| TEXAS INSTRUMENTS INCORPORATED
| Standard Linear and Logic Group
| IBIS Model of SN74AUC16373
| 16-BIT TRANSPARENT D-TYPE LATCH WITH 3-STATE OUTPUTS
| This file contains package information for the following:
|  TSSOP 48-pin (DGG) package as [Component] AUC16373_DGG
|   TVSOP 48-pin (DGV) package as [Component] AUC16373_DGV
|   VFBGA 56-pin (GQL) package as [Component] AUC16373_GQL
| This device can be powered at the following Vccs:
|  2.5 volt Vcc
|  1.8 volt Vcc
|  1.5 volt Vcc
|  1.2 volt Vcc
|  0.8 volt Vcc
| This file provides unique models under the [Model Selector] for each Vcc.
| For operation at a specific Vcc, select the appropriate model after each
| [Model Selector] keyword.
[IBIS Ver]   3.2
[Comment char]  |_char
[File Name]   sn74auc16373.ibs
[File Rev]   1.1 | x_die
[Date]   June 20, 2002
[Source]   Data created from TI-SPICE simulations at TI-SLL.
[Notes]   The following is an IBIS list for the AUC16373.
   Please contact sllibis@ti.com with questions and
   comments concerning SLL IBIS models.
   -The waveforms for the AUC16373_OUT Power Clamp ,Pullup, and
   Pulldown are caused by the circuitry that helps reduce
   overshoot and undershoot in transmission lines (EMI).
   These waveforms are norimal for this particular design.
   -Power clamp data deleted as there is no power-clamp diode.
   -End point warning due to AC and DC mismatch.
[Disclaimer] Property of Texas Instruments Incorporated.  Unauthorized
   reproduction and/or distribution is strictly prohibited.
   This product is protected under copyright law.
   Created  2002, (C) Copyright  2002, Texas Instruments
   Incorporated, All Rights Reserved
   UNLESS THERE IS A SIGNED, WRITTEN AGREEMENT TO THE
   CONTRARY, TEXAS INSTRUMENTS (TI) IS PROVIDING THE IBIS
   MODELS  AND WITHOUT ANY WARRANTY, EXPRESSED OR
   IMPLIED.  TI assumes no liability for:
   1) the accuracy of the IBIS models provided to your
   company;
   2) the proper functioning of these IBIS Models in your
   design or for any resulting applications; or
   3) infringement of patents, copyrights or intellectual
   property rights resulting from your use of these IBIS
   models.
   TI provides IBIS Models as a service to our customers.
   You and your company shall not distribute, sell or give
   these models to anyone else without prior written
   permission from TI.
   TI reserves the right to make changes to our products or
   to discontinue any semiconductor product or service
   without notice, and advises our customers to obtain the
   latest version of relevant information to verify, before
   placing orders, that the information being relied on is
   current.
   Please be aware that your receipt and use of the IBIS
   information provided shall serve as acceptance of these
   terms and conditions.  If you do not accept these terms,
   you should return or destroy the IBIS models and any
   other accompanying information immediately.
| Component AUC16373_DGG 48-pin TSSOP
[Component]   AUC16373_DGG
[Manufacturer]   Texas Instruments, Inc.
[Package]
|   typ   min   max
R_pkg   6.200e-02   5.000e-02   7.800e-02
L_pkg   3.527e-09   3.128e-09   4.255e-09
C_pkg   5.300e-13   4.170e-13   6.850e-13
[Pin]   signal_name   model_name   R_pin   L_pin   C_pin
1   1NOE   AUC16373_OEIN   5.000e-02   4.250e-09   6.710e-13
2   1Q1   AUC16373_OUT   5.700e-02   3.956e-09   6.740e-13
3   1Q2   AUC16373_OUT   7.100e-02   3.922e-09   6.190e-13
4   GND   GND   7.800e-02   3.841e-09   6.180e-13
5   1Q3   AUC16373_OUT   5.600e-02   3.535e-09   5.550e-13
6   1Q4   AUC16373_OUT   5.800e-02   3.464e-09   5.030e-13
7   VCC   POWER   6.000e-02   3.362e-09   4.980e-13
8   1Q5   AUC16373_OUT   6.100e-02   3.293e-09   4.620e-13
9   1Q6   AUC16373_OUT   6.300e-02   3.240e-09   4.550e-13
10   GND   GND   6.300e-02   3.175e-09   4.420e-13
11   1Q7   AUC16373_OUT   6.400e-02   3.153e-09   4.290e-13
12   1Q8   AUC16373_OUT   6.500e-02   3.128e-09   4.180e-13
13   2Q1   AUC16373_OUT   6.500e-02   3.128e-09   4.180e-13
14   2Q2   AUC16373_OUT   6.400e-02   3.154e-09   4.290e-13
15   GND   GND   6.300e-02   3.174e-09   4.420e-13
16   2Q3   AUC16373_OUT   6.300e-02   3.241e-09   4.550e-13
17   2Q4   AUC16373_OUT   6.100e-02   3.293e-09   4.620e-13
18   VCC   POWER   6.000e-02   3.362e-09   4.970e-13
19   2Q5   AUC16373_OUT   5.800e-02   3.464e-09   5.030e-13
20   2Q6   AUC16373_OUT   5.600e-02   3.537e-09   5.600e-13
21   GND   GND   7.700e-02   3.839e-09   6.260e-13
22   2Q7   AUC16373_OUT   7.100e-02   3.917e-09   6.270e-13
23   2Q8   AUC16373_OUT   5.800e-02   3.955e-09   6.850e-13
24   2NOE   AUC16373_OEIN   5.200e-02   4.255e-09   6.790e-13
25   2LE   AUC16373_LEIN   5.100e-02   4.254e-09   6.760e-13
26   2D8   AUC16373_IN   5.800e-02   3.957e-09   6.790e-13
27   2D7   AUC16373_IN   7.100e-02   3.920e-09   6.210e-13
28   GND   GND   7.800e-02   3.843e-09   6.220e-13
29   2D6   AUC16373_IN   5.600e-02   3.539e-09   5.600e-13
30   2D5   AUC16373_IN   5.800e-02   3.466e-09   5.030e-13
31   VCC   POWER   6.000e-02   3.363e-09   4.970e-13
32   2D4   AUC16373_IN   6.100e-02   3.294e-09   4.620e-13
33   2D3   AUC16373_IN   6.300e-02   3.241e-09   4.540e-13
34   GND   GND   6.300e-02   3.175e-09   4.410e-13
35   2D2   AUC16373_IN   6.400e-02   3.153e-09   4.290e-13
36   2D1   AUC16373_IN   6.500e-02   3.129e-09   4.170e-13
37   1D8   AUC16373_IN   6.500e-02   3.129e-09   4.170e-13
38   1D7   AUC16373_IN   6.400e-02   3.152e-09   4.290e-13
39   GND   GND   6.400e-02   3.176e-09   4.410e-13
40   1D6   AUC16373_IN   6.300e-02   3.241e-09   4.540e-13
41   1D5   AUC16373_IN   6.100e-02   3.293e-09   4.620e-13
42   VCC   POWER   6.000e-02   3.363e-09   4.970e-13
43   1D4   AUC16373_IN   5.800e-02   3.464e-09   5.030e-13
44   1D3   AUC16373_IN   5.600e-02   3.534e-09   5.610e-13
45   GND   GND   7.800e-02   3.841e-09   6.260e-13
46   1D2   AUC16373_IN   7.100e-02   3.920e-09   6.220e-13
47   1D1   AUC16373_IN   5.700e-02   3.955e-09   6.770e-13
48   1LE   AUC16373_LEIN   5.100e-02   4.252e-09   6.720e-13
| Component AUC16373_DGV 48-pin TVSOP
[Component]   AUC16373_DGV
[Manufacturer]   Texas Instruments, Inc.
[Package]
|   typ   min   max
R_pkg   7.000e-02   4.900e-02   8.500e-02
L_pkg   3.013e-09   2.743e-09   3.408e-09
C_pkg   3.710e-13   2.940e-13   5.110e-13
[Pin]   signal_name   model_name   R_pin   L_pin   C_pin
1   1NOE   AUC16373_OEIN   4.900e-02   3.393e-09   4.970e-13
2   1Q1   AUC16373_OUT   6.000e-02   3.250e-09   5.020e-13
3   1Q2   AUC16373_OUT   7.700e-02   3.310e-09   4.510e-13
4   GND   GND   8.500e-02   3.299e-09   4.040e-13
5   1Q3   AUC16373_OUT   8.300e-02   3.136e-09   3.600e-13
6   1Q4   AUC16373_OUT   7.700e-02   3.019e-09   3.630e-13
7   VCC   POWER   6.500e-02   2.882e-09   3.490e-13
8   1Q5   AUC16373_OUT   6.600e-02   2.829e-09   3.140e-13
9   1Q6   AUC16373_OUT   6.700e-02   2.796e-09   3.140e-13
10   GND   GND   6.900e-02   2.754e-09   3.080e-13
11   1Q7   AUC16373_OUT   7.000e-02   2.753e-09   3.010e-13
12   1Q8   AUC16373_OUT   7.100e-02   2.745e-09   2.940e-13
13   2Q1   AUC16373_OUT   7.000e-02   2.744e-09   2.940e-13
14   2Q2   AUC16373_OUT   7.000e-02   2.754e-09   3.010e-13
15   GND   GND   6.900e-02   2.754e-09   3.080e-13
16   2Q3   AUC16373_OUT   6.700e-02   2.796e-09   3.140e-13
17   2Q4   AUC16373_OUT   6.600e-02   2.829e-09   3.140e-13
18   VCC   POWER   6.500e-02   2.883e-09   3.500e-13
19   2Q5   AUC16373_OUT   7.500e-02   3.014e-09   3.630e-13
20   2Q6   AUC16373_OUT   8.000e-02   3.128e-09   3.580e-13
21   GND   GND   8.400e-02   3.295e-09   4.030e-13
22   2Q7   AUC16373_OUT   7.800e-02   3.311e-09   4.520e-13
23   2Q8   AUC16373_OUT   6.200e-02   3.259e-09   5.010e-13
24   2NOE   AUC16373_OEIN   5.200e-02   3.404e-09   4.960e-13
25   2LE   AUC16373_OEIN   5.300e-02   3.397e-09   5.050e-13
26   2D8   AUC16373_IN   6.200e-02   3.249e-09   5.110e-13
27   2D7   AUC16373_IN   7.700e-02   3.308e-09   4.530e-13
28   GND   GND   8.200e-02   3.289e-09   4.030e-13
29   2D6   AUC16373_IN   7.800e-02   3.121e-09   3.590e-13
30   2D5   AUC16373_IN   7.400e-02   3.010e-09   3.630e-13
31   VCC   POWER   6.500e-02   2.883e-09   3.490e-13
32   2D4   AUC16373_IN   6.700e-02   2.829e-09   3.140e-13
33   2D3   AUC16373_IN   6.700e-02   2.795e-09   3.140e-13
34   GND   GND   6.900e-02   2.753e-09   3.070e-13
35   2D2   AUC16373_IN   7.000e-02   2.753e-09   3.010e-13
36   2D1   AUC16373_IN   7.000e-02   2.743e-09   2.940e-13
37   1D8   AUC16373_IN   7.000e-02   2.743e-09   2.940e-13
38   1D7   AUC16373_IN   7.000e-02   2.753e-09   3.010e-13
39   GND   GND   6.900e-02   2.754e-09   3.070e-13
40   1D6   AUC16373_IN   6.800e-02   2.797e-09   3.140e-13
41   1D5   AUC16373_IN   6.700e-02   2.830e-09   3.140e-13
42   VCC   POWER   6.400e-02   2.880e-09   3.490e-13
43   1D4   AUC16373_IN   7.200e-02   3.004e-09   3.620e-13
44   1D3   AUC16373_IN   7.800e-02   3.121e-09   3.590e-13
45   GND   GND   8.400e-02   3.296e-09   4.030e-13
46   1D2   AUC16373_IN   7.700e-02   3.308e-09   4.510e-13
47   1D1   AUC16373_IN   6.200e-02   3.258e-09   4.990e-13
48   1LE   AUC16373_OEIN   5.300e-02   3.408e-09   4.940e-13
|   VFBGA PACKAGE (GQL)
[Component]   AUC16373_GQL
[manufacturer]   Texas Instruments, Inc.
[Package]
|   typ   min   max
R_pkg   0.065   0.035   0.097
L_pkg   1.952nH   1.000nH   3.191nH
C_pkg   0.283pF   0.162pF   0.434pF
[Pin] signal_name   model_name   R_pin   L_pin   C_pin
A3   NC   NC   0.036   1.004nH   0.176pF
A2   NC   NC   0.04   1.191nH   0.186pF
A1   1NOE   AUC16373_OEIN   0.047   1.411nH   0.209pF
B3   GND   GND   0.097   3.191nH   0.434pF
B2   1Q1   AUC16373_OUT   0.074   2.213nH   0.329pF
B1   1Q2   AUC16373_OUT   0.06   1.712nH   0.243pF
C3   VCC   POWER   0.085   2.691nH   0.368pF
C2   1Q3   AUC16373_OUT   0.074   2.16nH   0.315pF
C1   1Q4   AUC16373_OUT   0.06   1.666nH   0.247pF
D2   1Q5   AUC16373_OUT   0.074   2.121nH   0.313pF
D3   GND   GND   0.091   2.924nH   0.397pF
D1   1Q6   AUC16373_OUT   0.06   1.619nH   0.245pF
E2   1Q7   AUC16373_OUT   0.069   2.031nH   0.288pF
E1   1Q8   AUC16373_OUT   0.06   1.583nH   0.22pF
F1   2Q1   AUC16373_OUT   0.06   1.578nH   0.22pF
F2   2Q2   AUC16373_OUT   0.069   2.017nH   0.286pF
G1   2Q3   AUC16373_OUT   0.06   1.594nH   0.241pF
G3   GND   GND   0.092   2.917nH   0.397pF
G2   2Q4   AUC16373_OUT   0.075   2.114nH   0.315pF
H1   2Q5   AUC16373_OUT   0.06   1.632nH   0.247pF
H2   2Q6   AUC16373_OUT   0.07   2.074nH   0.307pF
H3   VCC   POWER   0.086   2.664nH   0.365pF
J1   2Q7   AUC16373_OUT   0.06   1.689nH   0.249pF
J2   2Q8   AUC16373_OUT   0.066   2.152nH   0.332pF
J3   GND   GND   0.087   3.118nH   0.423pF
K1   2NOE   AUC16373_OEIN   0.038   1.303nH   0.2pF
K2   NC   NC   0.035   1.176nH   0.183pF
K3   NC   NC   0.035   1.007nH   0.162pF
K4   NC   NC   0.035   1nH   0.162pF
K5   NC   NC   0.035   1.154nH   0.18pF
K6   2LE   AUC16373_LEIN   0.041   1.352nH   0.204pF
J4   GND   GND   0.088   3.137nH   0.43pF
J5   2D8   AUC16373_IN   0.074   2.218nH   0.334pF
J6   2D7   AUC16373_IN   0.06   1.683nH   0.25pF
H4   VCC   POWER   0.085   2.658nH   0.372pF
H5   2D6   AUC16373_IN   0.075   2.149nH   0.321pF
H6   2D5   AUC16373_IN   0.06   1.627nH   0.248pF
G5   2D4   AUC16373_IN   0.075   2.113nH   0.314pF
G4   GND   GND   0.092   2.922nH   0.396pF
G6   2D3   AUC16373_IN   0.06   1.594nH   0.242pF
F5   2D2   AUC16373_IN   0.069   2.016nH   0.288pF
F6   2D1   AUC16373_IN   0.06   1.58nH   0.221pF
E6   1D8   AUC16373_IN   0.06   1.582nH   0.22pF
E5   1D7   AUC16373_IN   0.069   2.026nH   0.289pF
D6   1D6   AUC16373_IN   0.06   1.61nH   0.245pF
D4   GND   GND   0.092   2.933nH   0.396pF
D5   1D5   AUC16373_IN   0.075   2.126nH   0.311pF
C6   1D4   AUC16373_IN   0.06   1.641nH   0.245pF
C5   1D3   AUC16373_IN   0.073   2.168nH   0.319pF
C4   VCC   POWER   0.086   2.675nH   0.362pF
B6   1D2   AUC16373_IN   0.06   1.688nH   0.243pF
B5   1D1   AUC16373_IN   0.075   2.281nH   0.333pF
B4   GND   GND   0.095   3.168nH   0.424pF
A6   1LE   AUC16373_LEIN   0.045   1.418nH   0.209pF
A5   NC   NC   0.039   1.216nH   0.19pF
A4   NC   NC   0.037   1.029nH   0.179pF
| Model AUC16373_LEIN
[Model Selector]   AUC16373_LEIN
AUC16373_LEIN_25   2.5 volt Vcc
AUC16373_LEIN_18   1.8 volt Vcc
AUC16373_LEIN_15A   1.5 volt Vcc
AUC16373_LEIN_12   1.2 volt Vcc
AUC16373_LEIN_08   0.8 volt Vcc
| Model AUC16373_IN
[Model Selector]   AUC16373_IN
AUC16373_IN_25   2.5 volt Vcc
AUC16373_IN_18   1.8 volt Vcc
AUC16373_IN_15A   1.5 volt Vcc
AUC16373_IN_12   1.2 volt Vcc
AUC16373_IN_08   0.8 volt Vcc
| Model AUC16373_OEIN
[Model Selector]   AUC16373_OEIN
AUC16373_OEIN_25   2.5 volt Vcc
AUC16373_OEIN_18   1.8 volt Vcc
AUC16373_OEIN_15A   1.5 volt Vcc
AUC16373_OEIN_12   1.2 volt Vcc
AUC16373_OEIN_08   0.8 volt Vcc
| Model AUC16373_OUT
[Model Selector]   AUC16373_OUT
AUC16373_OUT_25   2.5 volt Vcc
AUC16373_OUT_18   1.8 volt Vcc
AUC16373_OUT_15A   1.5 volt Vcc
AUC16373_OUT_12   1.2 volt Vcc
AUC16373_OUT_08   0.8 volt Vcc
| Models and submodels in the file (20): AUC16373_LEIN_25 (Input), AUC16373_LEIN_18 (Input), AUC16373_LEIN_15A (Input), AUC16373_LEIN_12 (Input), AUC16373_LEIN_08 (Input), AUC16373_IN_25 (Input), AUC16373_IN_18 (Input), AUC16373_IN_15A (Input), AUC16373_IN_12 (Input), AUC16373_IN_08 (Input), AUC16373_OEIN_25 (Input), AUC16373_OEIN_18 (Input), AUC16373_OEIN_15A (Input), AUC16373_OEIN_12 (Input), AUC16373_OEIN_08 (Input), AUC16373_OUT_25 (3-state), AUC16373_OUT_18 (3-state), AUC16373_OUT_15A (3-state), AUC16373_OUT_12 (3-state), AUC16373_OUT_08 (3-state)
